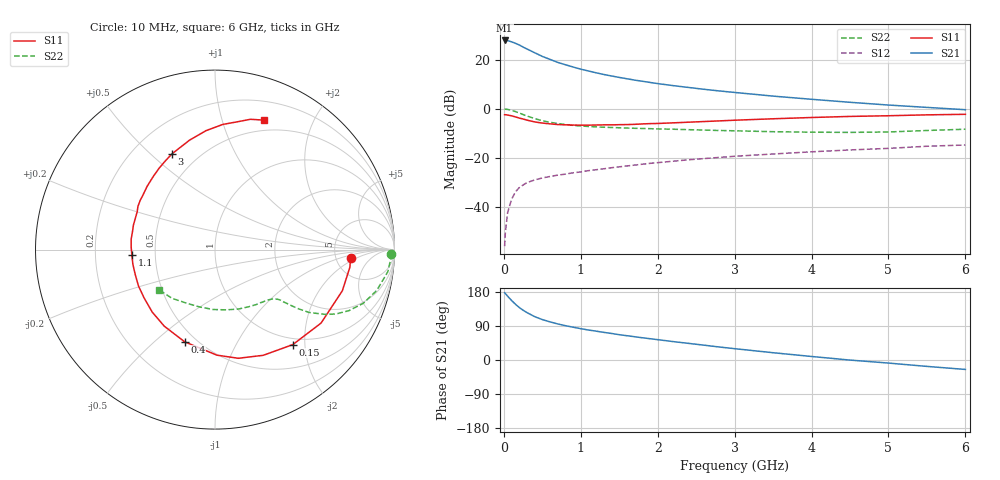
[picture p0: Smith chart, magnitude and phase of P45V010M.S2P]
! SIEMENS Small Signal Semiconductors
! BFP182
! Si NPN RF Bipolar Junction Transistor in SOT143
! VCE = 5 V  IC = 10 mA
! Common Emitter S-Parameters:  March  1996
# GHz  S  MA  R  50
!  f  S11  S21  S12  S22
! GHz  MAG  ANG  MAG  ANG  MAG  ANG  MAG  ANG
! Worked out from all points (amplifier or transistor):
!   36 points, 10 MHz to 6 GHz, reference 50 ohm
!   highest |S21| = 27.8 dB at 10 MHz (marker M1)
!   |S21| within 3 dB of that: start of sweep to 270.2 MHz
!   unconditionally stable (mu >= 1): 1.22 GHz to 5.397 GHz
!   at 250 MHz: K = 0.32, MSG = 28.1 dB, |S12| = -31.0 dB
!   at 1.4 GHz: K = 1.05, MAG = 17.3 dB, |S12| = -24.0 dB
!   at 6 GHz: K = 0.95, MSG = 7.2 dB, |S12| = -14.7 dB
!   lowest NFmin = 1.50 dB at 450 MHz
!   S11 on the Smith chart (normalised r, x): 10 MHz: 6.88, -1.49; 150 MHz: 0.88, -1.76; 400 MHz: 0.43, -0.63; 1.1 GHz: 0.37, -0.03; 3 GHz: 0.36, +0.59; 6 GHz: 0.39, +1.38
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0.01  0.7564 -3.5  24.57 177.4  0.0016 92.6  0.9823 -1.4
0.02  0.758 -7.4  24.55 175.5  0.0031 87.1  0.981 -2.9
0.05  0.7457 -17.9  24.39 168.2  0.0078 87.2  0.9708 -7.3
0.1  0.7189 -34.7  23.03 157.3  0.0143 71.7  0.9293 -14.2
0.15  0.6842 -50.7  21.53 147.3  0.0203 66.2  0.8786 -19.9
0.2  0.6473 -65.5  19.91 138.6  0.0248 61.3  0.8201 -24.5
0.25  0.6193 -77.9  18.03 131.3  0.0281 56.6  0.7638 -28.0
0.3  0.5881 -89.0  16.5 125.2  0.0314 53.1  0.7138 -30.4
0.4  0.5408 -108.2  13.83 114.5  0.0356 48.6  0.6318 -33.7
0.5  0.5119 -123.5  11.65 106.7  0.0391 45.8  0.5718 -35.3
0.6  0.4935 -135.1  10.12 100.6  0.0419 44.8  0.5307 -36.2
0.7  0.4779 -145.9  8.798 95.2  0.0446 44.3  0.5011 -36.8
0.9  0.4657 -162.3  7.085 86.6  0.0498 43.9  0.4595 -37.7
1.1  0.4641 -176.3  5.876 79.1  0.0551 44.6  0.4365 -39.1
1.5  0.4746 163.3  4.348 66.8  0.0658 44.5  0.4107 -42.9
1.8  0.492 150.8  3.634 58.7  0.0744 44.2  0.3974 -46.7
2.2  0.5172 136.9  2.961 48.6  0.0858 42.8  0.3836 -52.8
3  0.5851 114.1  2.15 29.9  0.108 37.9  0.3566 -68.1
3.5  0.626 103.1  1.811 19.2  0.1202 34.2  0.3417 -79.3
4.5  0.6989 86.4  1.355 -0.2  0.1453 27.0  0.3307 -105.1
5.5  0.7523 74.8  1.067 -16.9  0.1728 19.9  0.3616 -131.3
6  0.772 69.1  0.957 -24.9  0.1833 15.3  0.3838 -144.0
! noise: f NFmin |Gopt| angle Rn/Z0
0.45  1.5  0.26  43  0.28
0.9  1.6  0.24  87  0.22
1.8  2.1  0.2  170  0.2
